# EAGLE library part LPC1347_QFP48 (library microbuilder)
LPC1347 - ARM Cortex M3 72MHz MCU Supply: 2.0-3.6V 12-bit 500kHz ADC Flash: 64KB EEPROM: 4KB SRAM: 8KB SRAM0 + 2KB SRAM1 + 2KB USB Temp: -40°C - 85°C
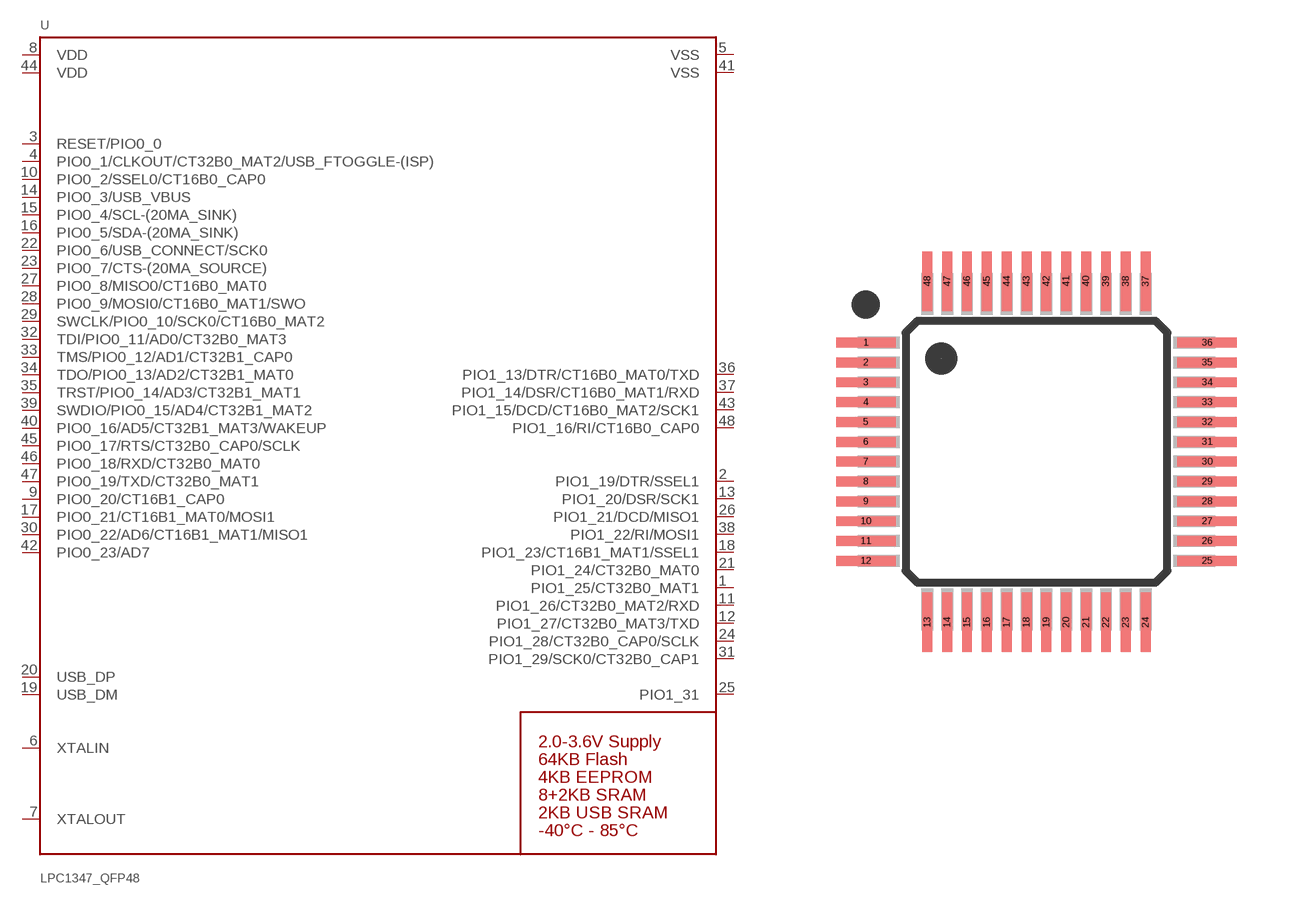
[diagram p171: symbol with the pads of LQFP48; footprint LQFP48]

Designator prefix U

## LPC1347_QFP48  [LQFP48]
1  PIO1_25/CT32B0_MAT1
2  PIO1_19/DTR/SSEL1
3  RESET/PIO0_0
4  PIO0_1/CLKOUT/CT32B0_MAT2/USB_FTOGGLE-(ISP)
5  VSS  pwr
6  XTALIN
7  XTALOUT
8  VDD  pwr
9  PIO0_20/CT16B1_CAP0
10  PIO0_2/SSEL0/CT16B0_CAP0
11  PIO1_26/CT32B0_MAT2/RXD
12  PIO1_27/CT32B0_MAT3/TXD
13  PIO1_20/DSR/SCK1
14  PIO0_3/USB_VBUS
15  PIO0_4/SCL-(20MA_SINK)
16  PIO0_5/SDA-(20MA_SINK)
17  PIO0_21/CT16B1_MAT0/MOSI1
18  PIO1_23/CT16B1_MAT1/SSEL1
19  USB_DM
20  USB_DP
21  PIO1_24/CT32B0_MAT0
22  PIO0_6/USB_CONNECT/SCK0
23  PIO0_7/CTS-(20MA_SOURCE)
24  PIO1_28/CT32B0_CAP0/SCLK
25  PIO1_31
26  PIO1_21/DCD/MISO1
27  PIO0_8/MISO0/CT16B0_MAT0
28  PIO0_9/MOSI0/CT16B0_MAT1/SWO
29  SWCLK/PIO0_10/SCK0/CT16B0_MAT2
30  PIO0_22/AD6/CT16B1_MAT1/MISO1
31  PIO1_29/SCK0/CT32B0_CAP1
32  TDI/PIO0_11/AD0/CT32B0_MAT3
33  TMS/PIO0_12/AD1/CT32B1_CAP0
34  TDO/PIO0_13/AD2/CT32B1_MAT0
35  TRST/PIO0_14/AD3/CT32B1_MAT1
36  PIO1_13/DTR/CT16B0_MAT0/TXD
37  PIO1_14/DSR/CT16B0_MAT1/RXD
38  PIO1_22/RI/MOSI1
39  SWDIO/PIO0_15/AD4/CT32B1_MAT2
40  PIO0_16/AD5/CT32B1_MAT3/WAKEUP
41  VSS  pwr
42  PIO0_23/AD7
43  PIO1_15/DCD/CT16B0_MAT2/SCK1
44  VDD  pwr
45  PIO0_17/RTS/CT32B0_CAP0/SCLK
46  PIO0_18/RXD/CT32B0_MAT0
47  PIO0_19/TXD/CT32B0_MAT1
48  PIO1_16/RI/CT16B0_CAP0

## Footprint LQFP48 (pad centres in mm)
smd 1.5 x 0.25: 1 -4.3,2.75; 2 -4.3,2.25; 3 -4.3,1.75; 4 -4.3,1.25; 5 -4.3,0.75; 6 -4.3,0.25; 7 -4.3,-0.25; 8 -4.3,-0.75; 9 -4.3,-1.25; 10 -4.3,-1.75; 11 -4.3,-2.25; 12 -4.3,-2.75; 25 4.3,-2.75; 26 4.3,-2.25; 27 4.3,-1.75; 28 4.3,-1.25; 29 4.3,-0.75; 30 4.3,-0.25; 31 4.3,0.25; 32 4.3,0.75; 33 4.3,1.25; 34 4.3,1.75; 35 4.3,2.25; 36 4.3,2.75
smd 0.25 x 1.5: 13 -2.75,-4.3; 14 -2.25,-4.3; 15 -1.75,-4.3; 16 -1.25,-4.3; 17 -0.75,-4.3; 18 -0.25,-4.3; 19 0.25,-4.3; 20 0.75,-4.3; 21 1.25,-4.3; 22 1.75,-4.3; 23 2.25,-4.3; 24 2.75,-4.3; 37 2.75,4.3; 38 2.25,4.3; 39 1.75,4.3; 40 1.25,4.3; 41 0.75,4.3; 42 0.25,4.3; 43 -0.25,4.3; 44 -0.75,4.3; 45 -1.25,4.3; 46 -1.75,4.3; 47 -2.25,4.3; 48 -2.75,4.3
